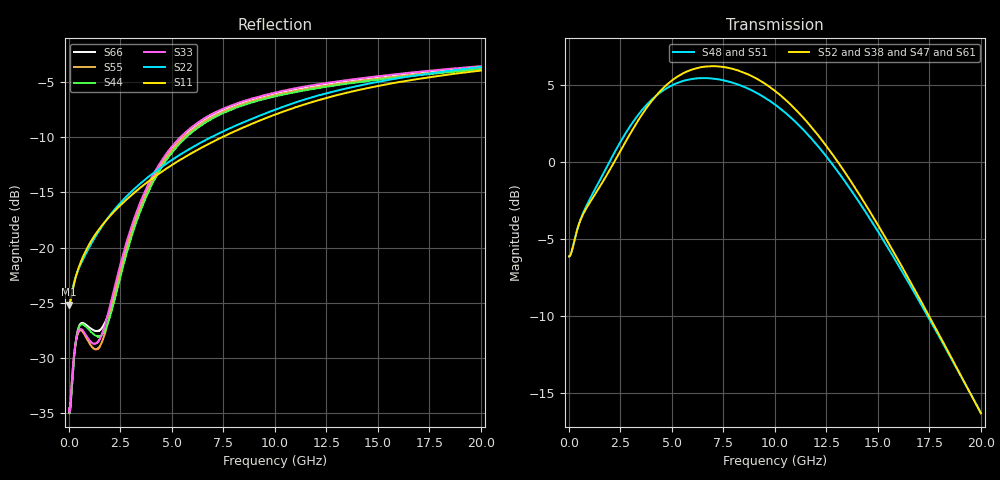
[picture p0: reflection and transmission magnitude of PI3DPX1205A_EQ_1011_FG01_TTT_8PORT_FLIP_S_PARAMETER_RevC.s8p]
! NPort=8 DATA=2000 NOISE=0 GROUPDELAY=0 COMPLEX_DATAFORMAT=POLAR
! NumOfBlock=1 NumOfParam=0
! .MODEL Smodel S TSTONEFILE=PI3DPX1205A_EQ_1011_FG01_TTT_8PORT_FLIP_S_PARAMETER_RevC.s8p TYPE=S
!  -- The above .MODEL line can be used for the S element in the netlist.
! The s parameter is extracted from the linear redriver, it is not bi-directional;
! only s(5,1)s(6,2)s(3,7)s(4,8) should be the insertion loss
!  Port definition:
!  Port1 = AIP
!  Port2 = AIN
!  Port3 = BOP
!  Port4 = BON
!  Port5 = AOP
!  Port6 = AON
!  Port7 = BIP
!  Port8 = BIN
# Hz S MA R  50
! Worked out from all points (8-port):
!   2000 points, 10 MHz to 20 GHz, reference 50 ohm
!   strongest paths, dB at 10 MHz, 5.01 GHz, 10.01 GHz, 15.01 GHz, 20 GHz:
!     S52: -6.1, 5.3, 4.6, -4.1, -16.3
!     S38: -6.1, 5.3, 4.6, -4.1, -16.3
!     S47: -6.1, 5.3, 4.6, -4.1, -16.3
!     S61: -6.1, 5.3, 4.6, -4.1, -16.3
!     S48: -6.1, 5.0, 3.7, -4.5, -16.3
!     S51: -6.1, 5.0, 3.7, -4.5, -16.3
!   lowest |S11| = -25.2 dB at 10 MHz (marker M1), VSWR 1.12, Z = 44.8 - j0.115 ohm
!   |S11| at or under -10 dB: start of sweep to 7.455 GHz
